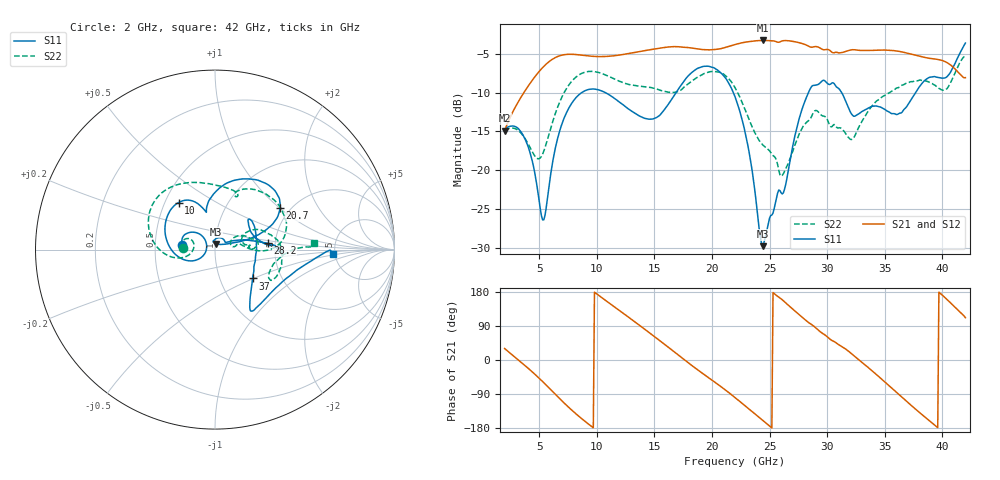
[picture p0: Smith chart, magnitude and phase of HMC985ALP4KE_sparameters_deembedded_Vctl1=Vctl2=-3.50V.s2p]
!s2p File: Measurements: S11, S21, S12, S22
# GHz S dB R 50.0
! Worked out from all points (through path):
!   401 points, 2 GHz to 42 GHz, reference 50 ohm
!   highest |S21| = -3.27 dB at 24.4 GHz (marker M1); lowest = -14.9 dB at 2 GHz (marker M2)
!   lowest |S11| = -29.8 dB at 24.4 GHz (marker M3), VSWR 1.07, Z = 50.7 + j3.2 ohm
!   |S11| at or under -10 dB: start of sweep to 8.683 GHz; 21.86 GHz to 28.37 GHz (6.518 GHz wide, 26 % of centre); 31.26 GHz to 37.68 GHz (6.418 GHz wide, 18.6 % of centre)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
!   |S22| runs from -20.8 to -5.1 dB; largest |S21 - S12| = 0.00067
!   S11 on the Smith chart (normalised r, x): 2 GHz: 0.69, +0.04; 10 GHz: 0.59, +0.35; 20.7 GHz: 1.77, +1.00; 28.2 GHz: 1.82, +0.14; 37 GHz: 1.43, -0.49; 42 GHz: 4.85, -0.40
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2  -14.68 171.6  -14.88 30.3  -14.88 30.3  -14.89 176.3
3.8  -16.05 141.9  -9.70 -15.4  -9.70 -15.4  -15.96 157.3
5.4  -26.38 178.0  -6.61 -59.9  -6.61 -59.9  -17.53 -172.8
6.8  -14.83 -161.9  -5.24 -102.5  -5.24 -102.6  -11.14 -174.7
8.7  -9.98 149.8  -5.17 -155.0  -5.17 -155.0  -7.51 149.4
10  -9.59 127.8  -5.34 174.3  -5.35 174.3  -7.34 128.1
13.1  -12.45 106.0  -4.88 105.3  -4.87 105.3  -9.03 83.8
15.4  -12.99 102.5  -4.28 52.7  -4.28 52.7  -9.62 67.2
17.8  -8.06 75.7  -4.17 -3.9  -4.17 -4.0  -9.02 68.3
20.7  -7.37 32.5  -4.35 -68.5  -4.35 -68.5  -7.39 22.4
22  -10.51 20.8  -3.80 -99.1  -3.80 -99.1  -9.35 2.8
23.1  -16.69 17.7  -3.45 -126.4  -3.44 -126.4  -12.99 -0.9
24.4  -29.77 76.5  -3.27 -159.1  -3.27 -159.1  -16.72 11.3
26.1  -23.04 35.6  -3.33 159.1  -3.33 159.1  -20.66 22.2
28.2  -10.61 6.8  -3.87 103.3  -3.87 103.3  -13.84 18.3
28.7  -9.13 0.6  -4.14 92.4  -4.15 92.4  -12.87 15.1
32.4  -13.03 27.9  -4.47 9.3  -4.47 9.2  -15.57 24.6
33.9  -11.76 40.5  -4.55 -28.5  -4.55 -28.5  -11.69 25.6
35.4  -12.50 12.7  -4.53 -68.6  -4.53 -68.7  -10.02 15.6
37  -11.58 -37.5  -4.92 -111.9  -4.92 -112.0  -8.72 2.7
39.6  -8.03 -53.9  -5.72 -178.4  -5.72 -178.5  -9.36 -28.2
42  -3.61 -2.0  -8.07 111.5  -8.07 111.5  -5.15 3.6
